|Texas Instruments Incorporated
|XWRL6844 Single-Chip 60GHz mmWave Sensor
[IBIS Ver]   5.0
[File name]   xwrl6844_fcbga207.ibs
[Date]   06/27/2024
[File Rev]   1.0
[Source]   Cadence SpeedXP Suite XtractIM 18.0.4.05011.160686   004
[Notes]   Revision History:
| Rev 1.0: 06/27/2024
| - Initial release of the model.
[Disclaimer]
| This model is designed as an aid for customers of Texas Instruments.
| TI and its licensors and suppliers make no warranties, either expressed
| or implied, with respect to this  model, including the warranties of
| merchantability or fitness for a particular purpose. The model is
| provided solely on an "as is" basis. The entire risk as to its quality
| and performance is with the customer.
| This model is subject to change without notice. Texas Instruments
| Incorporated is not responsible for updating this model.
[Copyright]
(C) Copyright 2021 Texas Instruments Incorporated.All rights reserved.
|  Component XA6844DBGANC 207-pin FCBGA - ANC0207 package
|  Part # XA6844DBGANC
[Component]   XA6844DBGANC
[Manufacturer]   Texas Instruments
[Package]   |207 FCBGA - ANC0207 package
|  variable   typ   min   max
R_pkg   0.14936   0.036665   0.28011
L_pkg   1.519e-9   4.001e-10   2.789e-9
C_pkg   4.347e-13   2.402e-13   6.324e-13
[Pin]   Signal_name   model_name   R_pin  L_pin  C_pin
A1   VSSA   GND   NA   NA   NA
A2   VSSA   GND   NA   NA   NA
A3   TX1   NC   NA   NA   NA
A4   VSSA   GND   NA   NA   NA
A5   TX2   NC   NA   NA   NA
A6   VSSA   GND   NA   NA   NA
A7   TX3   NC   NA   NA   NA
A8   VSSA   GND   NA   NA   NA
A9   TX4   NC   NA   NA   NA
A10   VSSA   GND   NA   NA   NA
A12   QSPI_dout   IO2   NA   NA   NA
A13   QSPI_cs_n   IO2   NA   NA   NA
A15   SPIA_mosi   IO2   NA   NA   NA
A16   SPIA_clk   IO2   NA   NA   NA
A17   VSS   GND   NA   NA   NA
B1   CLKM   NC   NA   NA   NA
B2   VSSA   GND   NA   NA   NA
B3   VSSA   GND   NA   NA   NA
B4   VSSA   GND   NA   NA   NA
B5   VSSA   GND   NA   NA   NA
B6   VSSA   GND   NA   NA   NA
B7   VSSA   GND   NA   NA   NA
B8   VSSA   GND   NA   NA   NA
B9   VSSA   GND   NA   NA   NA
B10   VSSA   GND   NA   NA   NA
B11   QSPI_qdin1   IO2   NA   NA   NA
B12   QSPI_qdin0   IO2   NA   NA   NA
B13   QSPI_din   IO2   NA   NA   NA
B14   QSPI_clk   IO2   NA   NA   NA
B15   SPIA_miso   IO2   NA   NA   NA
B16   VSS   GND   NA   NA   NA
B17   SPIA_cs0_n   IO2   NA   NA   NA
C1   VSSA   GND   NA   NA   NA
C2   VSSA   GND   NA   NA   NA
C16   HOST_CLK_req   IO2   NA   NA   NA
C17   PMIC_CLKOUT   IO2   NA   NA   NA
D1   CLKP   NC   NA   NA   NA
D2   VSSA   GND   NA   NA   NA
D3   VIOIN_18CLK   POWER   NA   NA   NA
D5   VDDA_10RF   POWER   NA   NA   NA
D6   VDDA_10RF   POWER   NA   NA   NA
D7   VDDA_10RF   POWER   NA   NA   NA
D8   VDDA_12RF   POWER   NA   NA   NA
D9   VDDA_12RF   POWER   NA   NA   NA
D10   VDDA_12RF   POWER   NA   NA   NA
D16   VSS   GND   NA   NA   NA
D17   VIOIN   POWER   NA   NA   NA
E1   VSSA   GND   NA   NA   NA
E2   VSSA   GND   NA   NA   NA
E7   VSSA   GND   NA   NA   NA
E8   VSSA   GND   NA   NA   NA
E9   VSSA   GND   NA   NA   NA
E10   VSS   GND   NA   NA   NA
E11   VSS   GND   NA   NA   NA
E12   VSS   GND   NA   NA   NA
E13   VDD   POWER   NA   NA   NA
E14   VDD   POWER   NA   NA   NA
E16   VSS   GND   NA   NA   NA
F1   VSSA   GND   NA   NA   NA
F2   VSSA   GND   NA   NA   NA
F3   VOUT_14SYNTH   NC   NA   NA   NA
F7   OSC_CLK_OUT   NC   NA   NA   NA
F8   VSSA   GND   NA   NA   NA
F9   VDD   POWER   NA   NA   NA
F10   VDD   POWER   NA   NA   NA
F11   VDD   POWER   NA   NA   NA
F12   VDD   POWER   NA   NA   NA
F13   VDD   POWER   NA   NA   NA
F14   VDD   POWER   NA   NA   NA
F16   GPIO_2   IO2   NA   NA   NA
F17   VIOIN_18   POWER   NA   NA   NA
G1   RX4   NC   NA   NA   NA
G2   VSSA   GND   NA   NA   NA
G3   VDDA_18VCO   POWER   NA   NA   NA
G7   VSSA   GND   NA   NA   NA
G8   VSSA   GND   NA   NA   NA
G9   VDD   POWER   NA   NA   NA
G10   VDD   POWER   NA   NA   NA
G11   VDD   POWER   NA   NA   NA
G12   VDD   POWER   NA   NA   NA
G13   VDD   POWER   NA   NA   NA
G14   VDD   POWER   NA   NA   NA
G16   LVDS_TXP0   ODF   NA   NA   NA
G17   LVDS_TXM0   ODF   NA   NA   NA
H1   VSSA   GND   NA   NA   NA
H2   VSSA   GND   NA   NA   NA
H7   VOUT_14APLL   NC   NA   NA   NA
H8   VSSA   GND   NA   NA   NA
H9   VDD   POWER   NA   NA   NA
H10   VDD   POWER   NA   NA   NA
H11   VDD   POWER   NA   NA   NA
H12   VDD   POWER   NA   NA   NA
H13   VDD   POWER   NA   NA   NA
H14   VDD   POWER   NA   NA   NA
H16   LVDS_CLKP   ODF   NA   NA   NA
J1   RX3   NC   NA   NA   NA
J2   VSSA   GND   NA   NA   NA
J7   VSSA   GND   NA   NA   NA
J8   VSSA   GND   NA   NA   NA
J9   VSS   GND   NA   NA   NA
J10   VSS   GND   NA   NA   NA
J11   VSS   GND   NA   NA   NA
J12   VSS   GND   NA   NA   NA
J13   VSS   GND   NA   NA   NA
J14   VSS   GND   NA   NA   NA
J16   VSS   GND   NA   NA   NA
J17   LVDS_CLKM   ODF   NA   NA   NA
K1   VSSA   GND   NA   NA   NA
K2   VSSA   GND   NA   NA   NA
K3   VBGAP   NC   NA   NA   NA
K5   VDDA_10RF   POWER   NA   NA   NA
K6   VSSA   GND   NA   NA   NA
K7   VSS   GND   NA   NA   NA
K8   VSS   GND   NA   NA   NA
K9   VSS   GND   NA   NA   NA
K10   VSS   GND   NA   NA   NA
K11   VSS   GND   NA   NA   NA
K12   VSS   GND   NA   NA   NA
K13   VSS   GND   NA   NA   NA
K14   VSS   GND   NA   NA   NA
K16   VIOIN_18LVDS   POWER   NA   NA   NA
K17   LVDS_FRCLKM   ODF   NA   NA   NA
L1   RX2   NC   NA   NA   NA
L2   VSSA   GND   NA   NA   NA
L5   VSSA   GND   NA   NA   NA
L6   VSSA   GND   NA   NA   NA
L7   VSS   GND   NA   NA   NA
L8   VSS   GND   NA   NA   NA
L9   VSS   GND   NA   NA   NA
L10   VSS   GND   NA   NA   NA
L11   VSS   GND   NA   NA   NA
L12   VSS   GND   NA   NA   NA
L13   VSS   GND   NA   NA   NA
L14   VSS   GND   NA   NA   NA
L16   LVDS_FRCLKP   ODF   NA   NA   NA
M1   VSSA   GND   NA   NA   NA
M2   VSSA   GND   NA   NA   NA
M4   VIN_18PM   POWER   NA   NA   NA
M5   VSSA   GND   NA   NA   NA
M6   VSSA   GND   NA   NA   NA
M7   VSS   GND   NA   NA   NA
M8   VSS   GND   NA   NA   NA
M9   VSS   GND   NA   NA   NA
M10   VSS   GND   NA   NA   NA
M11   VSS   GND   NA   NA   NA
M12   VSS   GND   NA   NA   NA
M13   VSS   GND   NA   NA   NA
M14   VSS   GND   NA   NA   NA
M16   LVDS_TXP1   ODF   NA   NA   NA
M17   LVDS_TXM1   ODF   NA   NA   NA
N1   RX1   NC   NA   NA   NA
N2   VSSA   GND   NA   NA   NA
N5   VSSA   GND   NA   NA   NA
N6   VSSA   GND   NA   NA   NA
N7   VSS   GND   NA   NA   NA
N8   VSS   GND   NA   NA   NA
N9   VSS   GND   NA   NA   NA
N10   VSS   GND   NA   NA   NA
N11   VSS   GND   NA   NA   NA
N12   VSS   GND   NA   NA   NA
N13   VSS   GND   NA   NA   NA
N14   VSS   GND   NA   NA   NA
N15   nERROR_OUT   IO2   NA   NA   NA
N16   I2C_scl   IO2   NA   NA   NA
N17   I2C_sda   IO2   NA   NA   NA
P1   VSSA   GND   NA   NA   NA
P2   VSSA   GND   NA   NA   NA
P15   rs232_tx   IO2   NA   NA   NA
P16   lvds_valid   IO2   NA   NA   NA
R1   VDDA_18BB   POWER   NA   NA   NA
R2   VDDA_18BB   POWER   NA   NA   NA
R4   VPP   POWER   NA   NA   NA
R10   UARTA_rx   IO1   NA   NA   NA
R11   CAN_FD_B_tx   IO1   NA   NA   NA
R14   rs232_rx   IO2   NA   NA   NA
R16   sys_reset_out  IO2   NA   NA   NA
R17   VIOIN_18   POWER   NA   NA   NA
T1   VSSA   GND   NA   NA   NA
T2   VSSA   GND   NA   NA   NA
T3   GPADC2   NC   NA   NA   NA
T4   GPADC1   NC   NA   NA   NA
T5   VDD   POWER   NA   NA   NA
T6   VNWA   POWER   NA   NA   NA
T7   VSS   GND   NA   NA   NA
T8   VSS   GND   NA   NA   NA
T9   VDD_SRAM   POWER   NA   NA   NA
T10   UARTA_tx   IO1   NA   NA   NA
T11   LIN_tx   IO1   NA   NA   NA
T12   TCK   IO1   NA   NA   NA
T13   TDO   IO1   NA   NA   NA
T14   TDI   IO1   NA   NA   NA
T15   TMS   IO1   NA   NA   NA
T16   VSS   GND   NA   NA   NA
T17   VIOIN   POWER   NA   NA   NA
U1   VSSA   GND   NA   NA   NA
U2   GPADC3   NC   NA   NA   NA
U3   GPADC4   NC   NA   NA   NA
U5   VDD   POWER   NA   NA   NA
U6   VIOIN   POWER   NA   NA   NA
U8   VIOIN_18   POWER   NA   NA   NA
U9   VDD_SRAM   POWER   NA   NA   NA
U10   NRESET   NC   NA   NA   NA
U12   CAN_FD_B_rx   IO1   NA   NA   NA
U13   LIN_rx   IO1   NA   NA   NA
U15   UARTA_rts   IO2   NA   NA   NA
U16   GPIO_5   IO2   NA   NA   NA
U17   VSS   GND   NA   NA   NA
[Diff Pin]  inv_pin  vdiff  tdelay_typ  tdelay_min  tdelay_max
   G16   G17   0.1   NA   NA   NA
   H16   J17   0.1   NA   NA   NA
   L16   K17   0.1   NA   NA   NA
   M16   M17   0.1   NA   NA   NA
| Model IO1
[Model Selector] IO1
|SC1 IS A SLEW RATE CONTROL PIN
|5% SUPPLY VARIATION MODES WITH 1.8V NOM SUPPLY
IO1_V_PUPDOFF_5P_SC1_1P8  Cell operated at 1.8(nom)
|IO1_V_PUPDOFF_5P_SC1_1P8; BUFFER WITH WEAK PULUP/PULLDOWN OFF AT 5% SUPPLY
|VARIATION WITH SC1=1 MEANING SLOW MODE OF OPERATION
IO1_V_PD_ON_5P_!SC1_1P8  Cell operated at 1.8(nom)
|IO1_V_PD_ON_5P_!SC1_1P8; BUFFER WITH WEAK_PULLDOWN_ON AT 5% SUPPLY
|VARIATION WITH SC1=0 MEANING FAST MODE OF OPERATION
IO1_V_PD_ON_5P_SC1_1P8  Cell operated at 1.8(nom)
|IO1_V_PD_ON_5P_SC1_1P8; BUFFER WITH WEAK_PULLDOWN_ON AT 5% SUPPLY
|VARIATION WITH SC1=1 MEANING SLOW MODE OF OPERATION
IO1_V_PU_ON_5P_!SC1_1P8  Cell operated at 1.8(nom)
|IO1_V_PU_ON_5P_!SC1_1P8; BUFFER WITH WEAK_PULLUP_ON AT 5% SUPPLY
|VARIATION WITH SC1=0 MEANING FAST MODE OF OPERATION
IO1_V_PUPDOFF_5P_!SC1_1P8  Cell operated at 1.8(nom)
|IO1_V_PUPDOFF_5P_!SC1_1P8; BUFFER WITH WEAK PULUP/PULLDOWN OFF AT 5% SUPPLY
|VARIATION WITH SC1=0 MEANING FAST MODE OF OPERATION
IO1_V_PU_ON_5P_SC1_1P8  Cell operated at 1.8(nom)
|IO1_V_PU_ON_5P_SC1_1P8; BUFFER WITH WEAK_PULLUP_ON AT 5% SUPPLY
|VARIATION WITH SC1=1 MEANING SLOW MODE OF OPERATION
|5% SUPPLY VARIATION MODES WITH 3.3V NOM SUPPLY
IO1_V_PUPDOFF_5P_SC1_3P3  Cell operated at 3.3(nom)
|IO1_V_PUPDOFF_5P_SC1_3P3; BUFFER WITH WEAK PULUP/PULLDOWN OFF AT 5% SUPPLY
|VARIATION WITH SC1=1 MEANING SLOW MODE OF OPERATION
IO1_V_PD_ON_5P_!SC1_3P3  Cell operated at 3.3(nom)
|IO1_V_PD_ON_5P_!SC1_3P3; BUFFER WITH WEAK_PULLDOWN_ON AT 5% SUPPLY
|VARIATION WITH SC1=0 MEANING FAST MODE OF OPERATION
IO1_V_PD_ON_5P_SC1_3P3  Cell operated at 3.3(nom)
|IO1_V_PD_ON_5P_SC1_3P3; BUFFER WITH WEAK_PULLDOWN_ON AT 5% SUPPLY
|VARIATION WITH SC1=1 MEANING SLOW MODE OF OPERATION
IO1_V_PU_ON_5P_!SC1_3P3  Cell operated at 3.3(nom)
|IO1_V_PU_ON_5P_!SC1_3P3; BUFFER WITH WEAK_PULLUP_ON AT 5% SUPPLY
|VARIATION WITH SC1=0 MEANING FAST MODE OF OPERATION
IO1_V_PUPDOFF_5P_!SC1_3P3  Cell operated at 3.3(nom)
|IO1_V_PUPDOFF_5P_!SC1_3P3; BUFFER WITH WEAK PULUP/PULLDOWN OFF AT 5% SUPPLY
|VARIATION WITH SC1=0 MEANING FAST MODE OF OPERATION
IO1_V_PU_ON_5P_SC1_3P3  Cell operated at 3.3(nom)
|IO1_V_PU_ON_5P_SC1_3P3; BUFFER WITH WEAK_PULLUP_ON AT 5% SUPPLY
|VARIATION WITH SC1=1 MEANING SLOW MODE OF OPERATION
| 10% SUPPLY VARIATION MODES WITH 1.8V NOM SUPPLY
IO1_V_PUPDOFF_10P_SC1_1P8  Cell operated at 1.8(nom)
|IO1_V_PUPDOFF_10P_SC1_1P8; BUFFER WITH WEAK PULUP/PULLDOWN OFF AT 10% SUPPLY
|VARIATION WITH SC1=1 MEANING SLOW MODE OF OPERATION
IO1_V_PD_ON_10P_!SC1_1P8  Cell operated at 1.8(nom)
|IO1_V_PD_ON_10P_!SC1_1P8; BUFFER WITH WEAK_PULLDOWN_ON AT 10% SUPPLY
|VARIATION WITH SC1=0 MEANING FAST MODE OF OPERATION
IO1_V_PD_ON_10P_SC1_1P8  Cell operated at 1.8(nom)
|IO1_V_PD_ON_10P_SC1_1P8; BUFFER WITH WEAK_PULLDOWN_ON AT 10% SUPPLY
|VARIATION WITH SC1=1 MEANING SLOW MODE OF OPERATION
IO1_V_PU_ON_10P_!SC1_1P8  Cell operated at 1.8(nom)
|IO1_V_PU_ON_10P_!SC1_1P8; BUFFER WITH WEAK_PULLUP_ON AT 10% SUPPLY
|VARIATION WITH SC1=0 MEANING FAST MODE OF OPERATION
IO1_V_PUPDOFF_10P_!SC1_1P8  Cell operated at 1.8(nom)
|IO1_V_PUPDOFF_10P_!SC1_1P8; BUFFER WITH WEAK PULUP/PULLDOWN OFF AT 10% SUPPLY
|VARIATION WITH SC1=0 MEANING FAST MODE OF OPERATION
IO1_V_PU_ON_10P_SC1_1P8  Cell operated at 1.8(nom)
|IO1_V_PU_ON_10P_SC1_1P8; BUFFER WITH WEAK_PULLUP_ON AT 10% SUPPLY
|VARIATION WITH SC1=1 MEANING SLOW MODE OF OPERATION
| 10% SUPPLY VARIATION MODES WITH 3.3V NOM SUPPLY
IO1_V_PUPDOFF_10P_SC1_3P3  Cell operated at 3.3(nom)
|IO1_V_PUPDOFF_10P_SC1_3P3; BUFFER WITH WEAK PULUP/PULLDOWN OFF AT 10% SUPPLY
|VARIATION WITH SC1=1 MEANING SLOW MODE OF OPERATION
IO1_V_PD_ON_10P_!SC1_3P3  Cell operated at 3.3(nom)
|IO1_V_PD_ON_10P_!SC1_3P3; BUFFER WITH WEAK_PULLDOWN_ON 10% SUPPLY
|VARIATION WITH SC1=0 MEANING FAST MODE OF OPERATION
IO1_V_PD_ON_10P_SC1_3P3  Cell operated at 3.3(nom)
|IO1_V_PD_ON_10P_SC1_3P3; BUFFER WITH WEAK_PULLDOWN_ON AT 10% SUPPLY
|VARIATION WITH SC1=1 MEANING SLOW MODE OF OPERATION
IO1_V_PU_ON_10P_!SC1_3P3  Cell operated at 3.3(nom)
|IO1_V_PU_ON_10P_!SC1_3P3; BUFFER WITH WEAK_PULLUP_ON AT 10% SUPPLY
|VARIATION WITH SC1=0 MEANING FAST MODE OF OPERATION
IO1_V_PUPDOFF_10P_!SC1_3P3  Cell operated at 3.3(nom)
|IO1_V_PUPDOFF_10P_!SC1_3P3; BUFFER WITH WEAK PULUP/PULLDOWN OFF AT 10% SUPPLY
|VARIATION WITH SC1=0 MEANING FAST MODE OF OPERATION
IO1_V_PU_ON_10P_SC1_3P3  Cell operated at 3.3(nom)
|IO1_V_PU_ON_10P_SC1_3P3; BUFFER WITH WEAK_PULLUP_ON AT 10% SUPPLY
|VARIATION WITH SC1=1 MEANING SLOW MODE OF OPERATION
| Model IO2
[Model Selector] IO2
|SC1 IS A SLEW RATE CONTROL PIN
|5% SUPPLY VARIATION MODES WITH 1.8V NOM SUPPLY
IO2_H_PUPDOFF_5P_SC1_1P8  Cell operated at 1.8(nom)
|IO2_H_PUPDOFF_5P_SC1_1P8; BUFFER WITH WEAK PULUP/PULLDOWN OFF AT 5% SUPPLY
|VARIATION WITH SC1=1 MEANING SLOW MODE OF OPERATION
IO2_H_PD_ON_5P_!SC1_1P8  Cell operated at 1.8(nom)
|IO2_H_PD_ON_5P_!SC1_1P8; BUFFER WITH WEAK_PULLDOWN_ON AT 5% SUPPLY
|VARIATION WITH SC1=0 MEANING FAST MODE OF OPERATION
IO2_H_PD_ON_5P_SC1_1P8  Cell operated at 1.8(nom)
|IO2_H_PD_ON_5P_SC1_1P8; BUFFER WITH WEAK_PULLDOWN_ON AT 5% SUPPLY
|VARIATION WITH SC1=1 MEANING SLOW MODE OF OPERATION
IO2_H_PU_ON_5P_!SC1_1P8  Cell operated at 1.8(nom)
|IO2_H_PU_ON_5P_!SC1_1P8; BUFFER WITH WEAK_PULLUP_ON AT 5% SUPPLY
|VARIATION WITH SC1=0 MEANING FAST MODE OF OPERATION
IO2_H_PUPDOFF_5P_!SC1_1P8  Cell operated at 1.8(nom)
|IO2_H_PUPDOFF_5P_!SC1_1P8; BUFFER WITH WEAK PULUP/PULLDOWN OFF AT 5% SUPPLY
|VARIATION WITH SC1=0 MEANING FAST MODE OF OPERATION
IO2_H_PU_ON_5P_SC1_1P8  Cell operated at 1.8(nom)
|IO2_H_PU_ON_5P_SC1_1P8; BUFFER WITH WEAK_PULLUP_ON AT 5% SUPPLY
|VARIATION WITH SC1=1 MEANING SLOW MODE OF OPERATION
|5% SUPPLY VARIATION MODES WITH 3.3V NOM SUPPLY
IO2_H_PUPDOFF_5P_SC1_3P3  Cell operated at 3.3(nom)
|IO2_H_PUPDOFF_5P_SC1_3P3; BUFFER WITH WEAK PULUP/PULLDOWN OFF AT 5% SUPPLY
|VARIATION WITH SC1=1 MEANING SLOW MODE OF OPERATION
IO2_H_PD_ON_5P_!SC1_3P3  Cell operated at 3.3(nom)
|IO2_H_PD_ON_5P_!SC1_3P3; BUFFER WITH WEAK_PULLDOWN_ON AT 5% SUPPLY
|VARIATION WITH SC1=0 MEANING FAST MODE OF OPERATION
IO2_H_PD_ON_5P_SC1_3P3  Cell operated at 3.3(nom)
|IO2_H_PD_ON_5P_SC1_3P3; BUFFER WITH WEAK_PULLDOWN_ON AT 5% SUPPLY
|VARIATION WITH SC1=1 MEANING SLOW MODE OF OPERATION
IO2_H_PU_ON_5P_!SC1_3P3  Cell operated at 3.3(nom)
|IO2_H_PU_ON_5P_!SC1_3P3; BUFFER WITH WEAK_PULLUP_ON AT 5% SUPPLY
|VARIATION WITH SC1=0 MEANING FAST MODE OF OPERATION
IO2_H_PUPDOFF_5P_!SC1_3P3  Cell operated at 3.3(nom)
|IO2_H_PUPDOFF_5P_!SC1_3P3; BUFFER WITH WEAK PULUP/PULLDOWN OFF AT 5% SUPPLY
|VARIATION WITH SC1=0 MEANING FAST MODE OF OPERATION
IO2_H_PU_ON_5P_SC1_3P3  Cell operated at 3.3(nom)
|IO2_H_PU_ON_5P_SC1_3P3; BUFFER WITH WEAK_PULLUP_ON AT 5% SUPPLY
|VARIATION WITH SC1=1 MEANING SLOW MODE OF OPERATION
| 10% SUPPLY VARIATION MODES WITH 1.8V NOM SUPPLY
IO2_H_PUPDOFF_10P_SC1_1P8  Cell operated at 1.8(nom)
|IO2_H_PUPDOFF_10P_SC1_1P8; BUFFER WITH WEAK PULUP/PULLDOWN OFF AT 10% SUPPLY
|VARIATION WITH SC1=1 MEANING SLOW MODE OF OPERATION
IO2_H_PD_ON_10P_!SC1_1P8  Cell operated at 1.8(nom)
|IO2_H_PD_ON_10P_!SC1_1P8; BUFFER WITH WEAK_PULLDOWN_ON AT 10% SUPPLY
|VARIATION WITH SC1=0 MEANING FAST MODE OF OPERATION
IO2_H_PD_ON_10P_SC1_1P8  Cell operated at 1.8(nom)
|IO2_H_PD_ON_10P_SC1_1P8; BUFFER WITH WEAK_PULLDOWN_ON AT 10% SUPPLY
|VARIATION WITH SC1=1 MEANING SLOW MODE OF OPERATION
IO2_H_PU_ON_10P_!SC1_1P8  Cell operated at 1.8(nom)
|IO2_H_PU_ON_10P_!SC1_1P8; BUFFER WITH WEAK_PULLUP_ON AT 10% SUPPLY
|VARIATION WITH SC1=0 MEANING FAST MODE OF OPERATION
IO2_H_PUPDOFF_10P_!SC1_1P8  Cell operated at 1.8(nom)
|IO2_H_PUPDOFF_10P_!SC1_1P8; BUFFER WITH WEAK PULUP/PULLDOWN OFF AT 10% SUPPLY
|VARIATION WITH SC1=0 MEANING FAST MODE OF OPERATION
IO2_H_PU_ON_10P_SC1_1P8  Cell operated at 1.8(nom)
|IO2_H_PU_ON_10P_SC1_1P8; BUFFER WITH WEAK_PULLUP_ON AT 10% SUPPLY
|VARIATION WITH SC1=1 MEANING SLOW MODE OF OPERATION
| 10% SUPPLY VARIATION MODES WITH 3.3V NOM SUPPLY
IO2_H_PUPDOFF_10P_SC1_3P3  Cell operated at 3.3(nom)
|IO2_H_PUPDOFF_10P_SC1_3P3; BUFFER WITH WEAK PULUP/PULLDOWN OFF AT 10% SUPPLY
|VARIATION WITH SC1=1 MEANING SLOW MODE OF OPERATION
IO2_H_PD_ON_10P_!SC1_3P3  Cell operated at 3.3(nom)
|IO2_H_PD_ON_10P_!SC1_3P3; BUFFER WITH WEAK_PULLDOWN_ON 10% SUPPLY
|VARIATION WITH SC1=0 MEANING FAST MODE OF OPERATION
IO2_H_PD_ON_10P_SC1_3P3  Cell operated at 3.3(nom)
|IO2_H_PD_ON_10P_SC1_3P3; BUFFER WITH WEAK_PULLDOWN_ON AT 10% SUPPLY
|VARIATION WITH SC1=1 MEANING SLOW MODE OF OPERATION
IO2_H_PU_ON_10P_!SC1_3P3  Cell operated at 3.3(nom)
|IO2_H_PU_ON_10P_!SC1_3P3; BUFFER WITH WEAK_PULLUP_ON AT 10% SUPPLY
|VARIATION WITH SC1=0 MEANING FAST MODE OF OPERATION
IO2_H_PUPDOFF_10P_!SC1_3P3  Cell operated at 3.3(nom)
|IO2_H_PUPDOFF_10P_!SC1_3P3; BUFFER WITH WEAK PULUP/PULLDOWN OFF AT 10% SUPPLY
|VARIATION WITH SC1=0 MEANING FAST MODE OF OPERATION
IO2_H_PU_ON_10P_SC1_3P3  Cell operated at 3.3(nom)
|IO2_H_PU_ON_10P_SC1_3P3; BUFFER WITH WEAK_PULLUP_ON AT 10% SUPPLY
|VARIATION WITH SC1=1 MEANING SLOW MODE OF OPERATION
| Model ODF
[Model Selector] ODF
ODF_MODE_10P_1P8  Cell operated at 1.8(nom)
|ODF_MODE_10P_1P8; LVDS DRIVER MODE WITH 10PER VDDS
ODF_MODE_5P_1P8  Cell operated at 1.8(nom)
[Define Package Model]   XA6844DBGANC
[Manufacturer]   TI
[OEM]   TI
[Description]   FCBGA
|[Number of Sections]   1
[Number of Pins]   64
[Pin Numbers]
|[Pin Name]  Net Number   Net Name   Net's All Pins
B1   | 1   CLKM   B1
D1   | 2   CLKP   D1
F7   | 3   OSC_CLK_OUT   F7
K3   | 4   VBGAP   K3
U5   | 5   VDD   U5
   |T5
   |H14
   |H13
   |H12
   |H11
   |H10
   |H9
   |G14
   |G13
   |G12
   |G11
   |G10
   |G9
   |F14
   |F13
   |F12
   |F11
   |F10
   |F9
   |E14
   |E13
K5   | 6   VDDA_10RF   K5
   |D7
   |D6
   |D5
D10   | 7   VDDA_12RF   D10
   |D9
   |D8
R2   | 8   VDDA_18BB   R2
   |R1
G3   | 9   VDDA_18VCO   G3
U9   | 10   VDD_SRAM   U9
   |T9
M4   | 11   VIN_18PM   M4
U6   | 12   VIOIN   U6
   |T17
   |D17
U8   | 13   VIOIN_18   U8
   |R17
   |F17
D3   | 14   VIOIN_18CLK   D3
K16   | 15   VIOIN_18LVDS   K16
T6   | 16   VNWA   T6
H7   | 17   VOUT_14APLL   H7
F3   | 18   VOUT_14SYNTH   F3
R4   | 19   VPP   R4
U12   | 20   CAN_FD_B_RX   U12
R11   | 21   CAN_FD_B_TX   R11
T4   | 22   GPADC1   T4
T3   | 23   GPADC2   T3
U2   | 24   GPADC3   U2
U3   | 25   GPADC4   U3
F16   | 26   GPIO_2   F16
U16   | 27   GPIO_5   U16
C16   | 28   HOST_CLK_REQ   C16
N16   | 29   I2C_SCL   N16
N17   | 30   I2C_SDA   N17
U13   | 31   LIN_RX   U13
T11   | 32   LIN_TX   T11
J17   | 33   LVDS_CLKM   J17
H16   | 34   LVDS_CLKP   H16
K17   | 35   LVDS_FRCLKM   K17
L16   | 36   LVDS_FRCLKP   L16
G17   | 37   LVDS_TXM0   G17
M17   | 38   LVDS_TXM1   M17
G16   | 39   LVDS_TXP0   G16
M16   | 40   LVDS_TXP1   M16
P16   | 41   LVDS_VALID   P16
N15   | 42   NERROR_OUT   N15
U10   | 43   NRESET   U10
C17   | 44   PMIC_CLKOUT   C17
B14   | 45   QSPI_CLK   B14
A13   | 46   QSPI_CS_N   A13
B13   | 47   QSPI_DIN   B13
A12   | 48   QSPI_DOUT   A12
B12   | 49   QSPI_QDIN0   B12
B11   | 50   QSPI_QDIN1   B11
R14   | 51   RS232_RX   R14
P15   | 52   RS232_TX   P15
A16   | 53   SPIA_CLK   A16
B17   | 54   SPIA_CS0_N   B17
B15   | 55   SPIA_MISO   B15
A15   | 56   SPIA_MOSI   A15
R16   | 57   SYS_RESET_OUT   R16
T12   | 58   TCK   T12
T14   | 59   TDI   T14
T13   | 60   TDO   T13
T15   | 61   TMS   T15
U15   | 62   UARTA_RTS   U15
R10   | 63   UARTA_RX   R10
T10   | 64   UARTA_TX   T10
[Model Data]
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[End Model Data]
[End Package Model]
| Models and submodels in the file (50): IO1_V_PUPDOFF_5P_SC1_1P8 (I/O), IO1_V_PD_ON_5P_!SC1_1P8 (I/O), IO1_V_PD_ON_5P_SC1_1P8 (I/O), IO1_V_PU_ON_5P_!SC1_1P8 (I/O), IO1_V_PUPDOFF_5P_!SC1_1P8 (I/O), IO1_V_PU_ON_5P_SC1_1P8 (I/O), IO1_V_PUPDOFF_5P_SC1_3P3 (I/O), IO1_V_PD_ON_5P_!SC1_3P3 (I/O), IO1_V_PD_ON_5P_SC1_3P3 (I/O), IO1_V_PU_ON_5P_!SC1_3P3 (I/O), IO1_V_PUPDOFF_5P_!SC1_3P3 (I/O), IO1_V_PU_ON_5P_SC1_3P3 (I/O), IO1_V_PUPDOFF_10P_SC1_1P8 (I/O), IO1_V_PD_ON_10P_!SC1_1P8 (I/O), IO1_V_PD_ON_10P_SC1_1P8 (I/O), IO1_V_PU_ON_10P_!SC1_1P8 (I/O), IO1_V_PUPDOFF_10P_!SC1_1P8 (I/O), IO1_V_PU_ON_10P_SC1_1P8 (I/O), IO1_V_PUPDOFF_10P_SC1_3P3 (I/O), IO1_V_PD_ON_10P_!SC1_3P3 (I/O), IO1_V_PD_ON_10P_SC1_3P3 (I/O), IO1_V_PU_ON_10P_!SC1_3P3 (I/O), IO1_V_PUPDOFF_10P_!SC1_3P3 (I/O), IO1_V_PU_ON_10P_SC1_3P3 (I/O), IO2_H_PUPDOFF_5P_SC1_1P8 (I/O), IO2_H_PD_ON_5P_!SC1_1P8 (I/O), IO2_H_PD_ON_5P_SC1_1P8 (I/O), IO2_H_PU_ON_5P_!SC1_1P8 (I/O), IO2_H_PUPDOFF_5P_!SC1_1P8 (I/O), IO2_H_PU_ON_5P_SC1_1P8 (I/O), IO2_H_PUPDOFF_5P_SC1_3P3 (I/O), IO2_H_PD_ON_5P_!SC1_3P3 (I/O), IO2_H_PD_ON_5P_SC1_3P3 (I/O), IO2_H_PU_ON_5P_!SC1_3P3 (I/O), IO2_H_PUPDOFF_5P_!SC1_3P3 (I/O), IO2_H_PU_ON_5P_SC1_3P3 (I/O), IO2_H_PUPDOFF_10P_SC1_1P8 (I/O), IO2_H_PD_ON_10P_!SC1_1P8 (I/O), IO2_H_PD_ON_10P_SC1_1P8 (I/O), IO2_H_PU_ON_10P_!SC1_1P8 (I/O), IO2_H_PUPDOFF_10P_!SC1_1P8 (I/O), IO2_H_PU_ON_10P_SC1_1P8 (I/O), IO2_H_PUPDOFF_10P_SC1_3P3 (I/O), IO2_H_PD_ON_10P_!SC1_3P3 (I/O), IO2_H_PD_ON_10P_SC1_3P3 (I/O), IO2_H_PU_ON_10P_!SC1_3P3 (I/O), IO2_H_PUPDOFF_10P_!SC1_3P3 (I/O), IO2_H_PU_ON_10P_SC1_3P3 (I/O), ODF_MODE_10P_1P8 (3-state), ODF_MODE_5P_1P8 (3-state)
